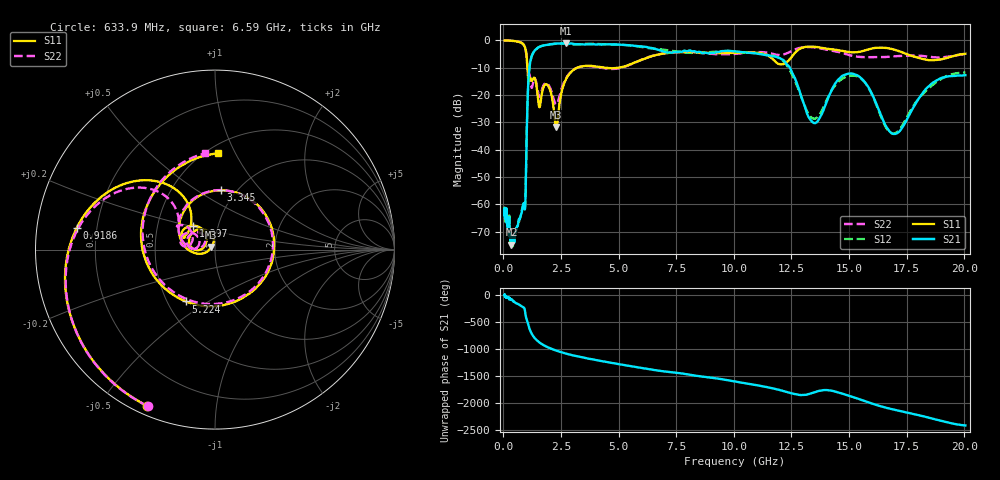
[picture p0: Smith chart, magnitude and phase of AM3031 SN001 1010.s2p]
# Hz S DB R 50
!freq MagS11 AngS11 MagS21 AngS21 MagS12 AngS12 MagS22 AngS22
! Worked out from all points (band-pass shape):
!   1601 points, 50 MHz to 20.05 GHz, reference 50 ohm
!   highest |S21| = -1.05 dB at 2.702 GHz (marker M1); lowest = -74.7 dB at 346.8 MHz (marker M2)
!   |S21| within 3 dB of the highest: 1.324 GHz to 6.923 GHz (5.599 GHz wide, 136 % of centre); 9.408 GHz to 10.09 GHz (682.5 MHz wide, 7 % of centre)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
!   lowest |S11| = -31.6 dB at 2.291 GHz (marker M3), VSWR 1.05, Z = 47.9 + j1.45 ohm
!   |S11| at or under -10 dB: 1.041 GHz to 3.193 GHz (2.152 GHz wide, 102 % of centre); 4.422 GHz to 4.969 GHz (546.5 MHz wide, 11.6 % of centre)
!   |S22| runs from -23.4 to 0.0 dB; largest |S21 - S12| = 0.067
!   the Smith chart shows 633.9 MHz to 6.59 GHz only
!   S11 on the Smith chart (normalised r, x): 633.9 MHz: 0.04, -0.65; 918.6 MHz: 0.12, +0.08; 1.397 GHz: 0.76, +0.21; 3.345 GHz: 0.85, +0.63; 5.224 GHz: 0.62, -0.40; 6.59 GHz: 0.57, +0.85
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5e7  -0.02 -8.6  -61.83 -16.3  -61.86 3.8  -0.04 -8.5
1.35947e8  -0.05 -23.1  -66.07 -37.4  -65.41 -36.3  -0.04 -23.0
3.468255e8  -0.13 -59.1  -74.72 -84.4  -73.79 -86.1  -0.12 -59.4
3.696318e8  -0.14 -63.1  -73.59 -89.8  -74.85 -92.0  -0.14 -63.5
6.339456e8  -0.45 -113.6  -67.12 -172.3  -66.71 -170.8  -0.45 -113.3
9.185894e8  -2.17 170.9  -61.24 99.0  -60.95 99.9  -2.18 172.6
1.005007e9  -5.79 131.7  -35.90 -86.5  -35.79 -87.9  -6.31 136.2
1.397468e9  -14.90 132.0  -3.37 -97.6  -3.39 -97.6  -14.57 150.9
1.691674e9  -18.44 178.7  -2.00 163.3  -1.96 163.1  -17.45 177.3
2.291401e9  -31.62 144.7  -1.13 49.9  -1.18 50.0  -23.42 152.7
2.702015e9  -14.38 166.8  -1.05 -3.5  -1.27 -3.5  -14.07 162.2
2.722335e9  -14.05 164.0  -1.07 -6.1  -1.27 -6.0  -13.77 160.1
3.345218e9  -9.57 84.3  -1.44 -68.7  -1.40 -66.5  -9.62 89.2
5.224365e9  -9.59 -119.2  -1.63 144.3  -1.64 144.5  -9.73 -130.0
6.590295e9  -5.41 88.4  -3.12 49.0  -3.04 52.7  -5.36 95.8
7.401857e9  -4.37 8.6  -4.29 7.0  -3.96 2.8  -4.34 26.7
8.728265e9  -4.45 -107.6  -4.46 -74.2  -4.40 -72.1  -4.72 -89.8
1.017731e10  -4.48 122.0  -4.12 -169.6  -4.18 -168.4  -4.84 119.4
1.151657e10  -5.70 -23.5  -5.44 89.2  -5.29 88.6  -4.58 -5.3
1.378533e10  -2.68 -178.0  -27.42 33.7  -26.23 29.9  -2.97 -159.4
1.63779e10  -2.62 16.8  -27.25 101.9  -27.73 104.3  -6.11 21.7
2.005e10  -4.90 41.3  -12.72 108.2  -11.73 108.0  -4.99 66.0
